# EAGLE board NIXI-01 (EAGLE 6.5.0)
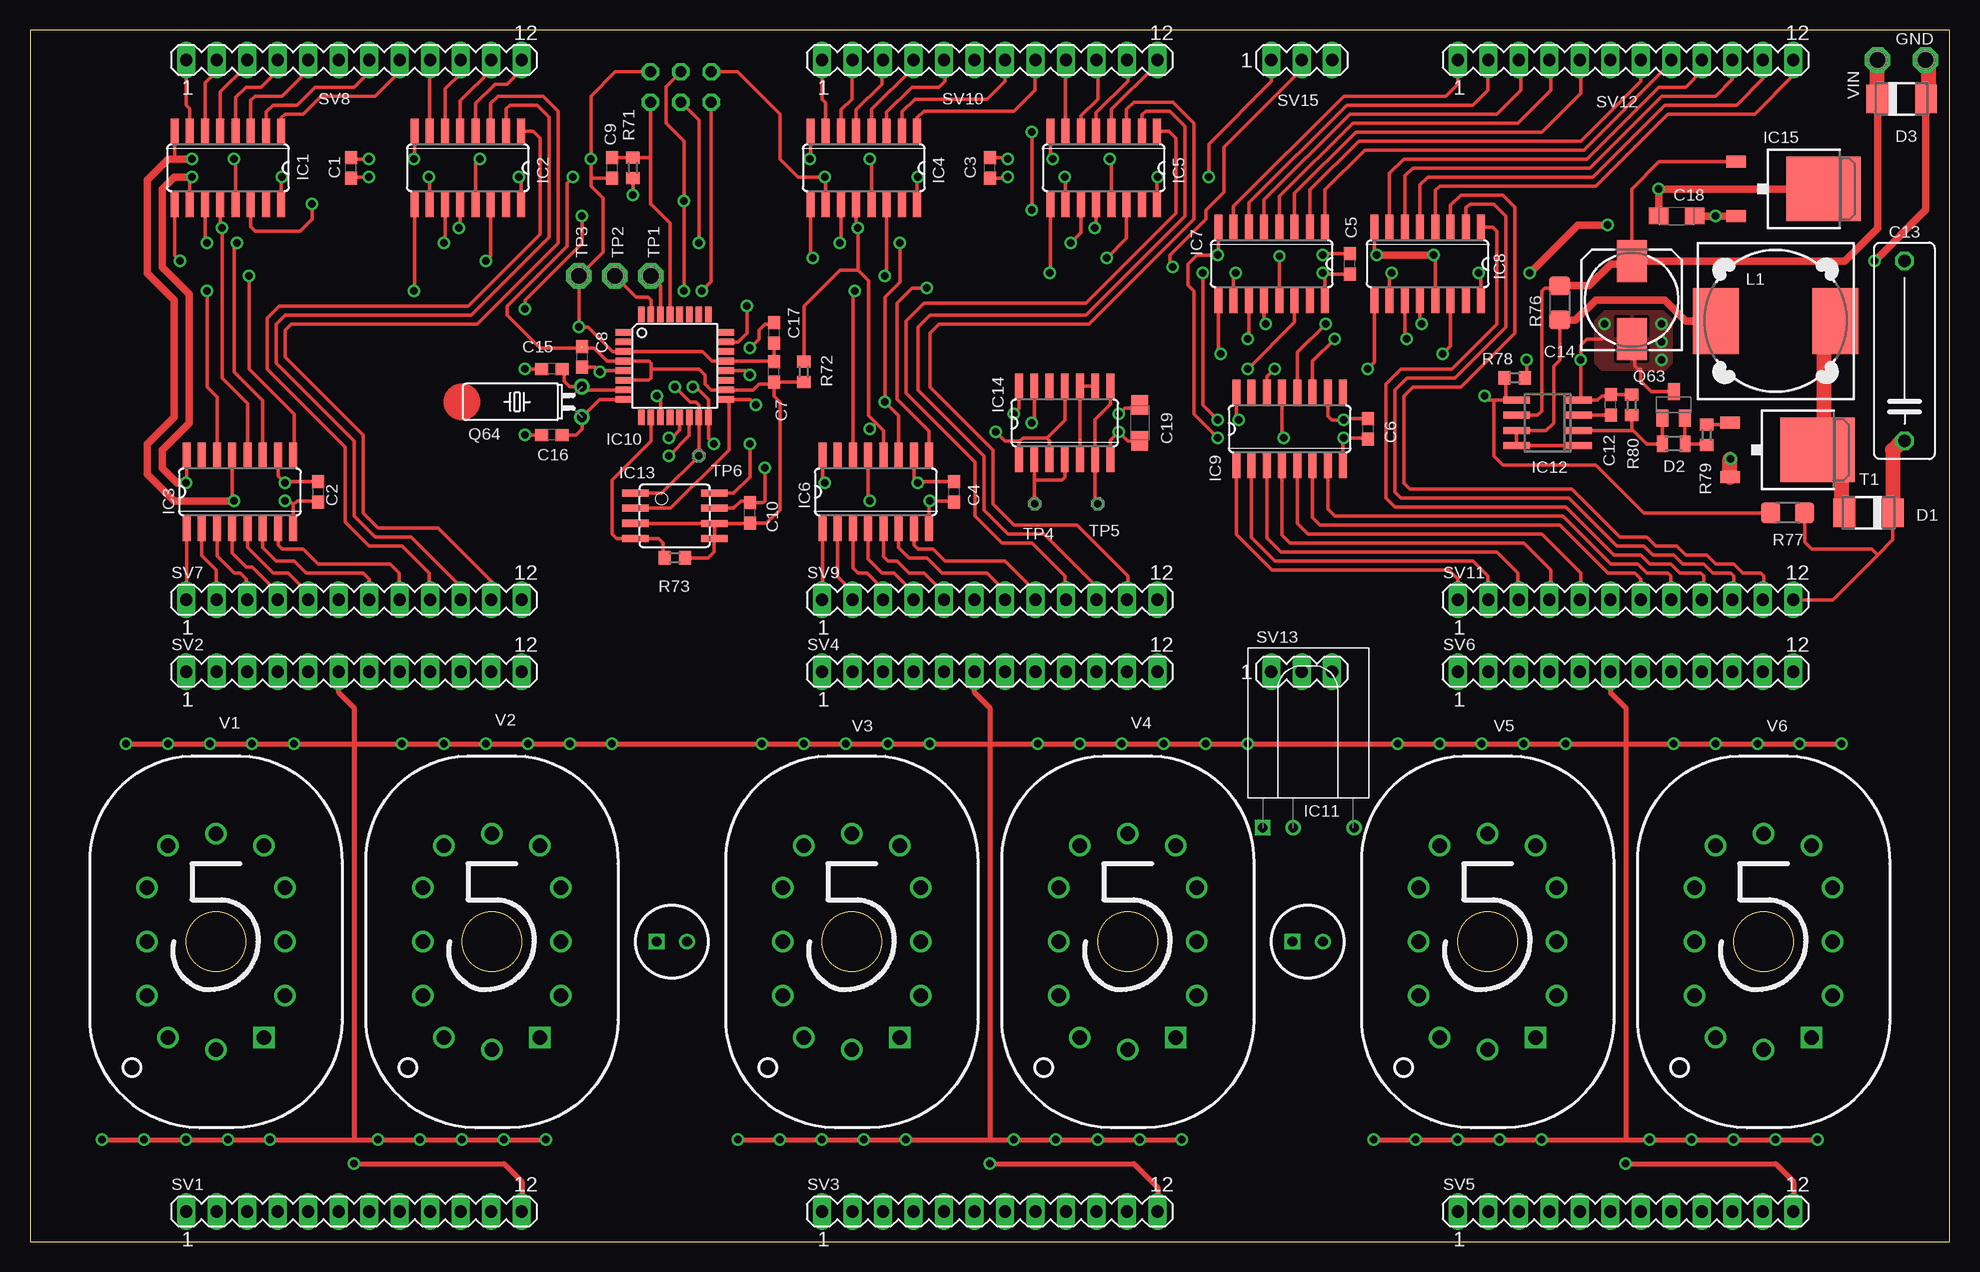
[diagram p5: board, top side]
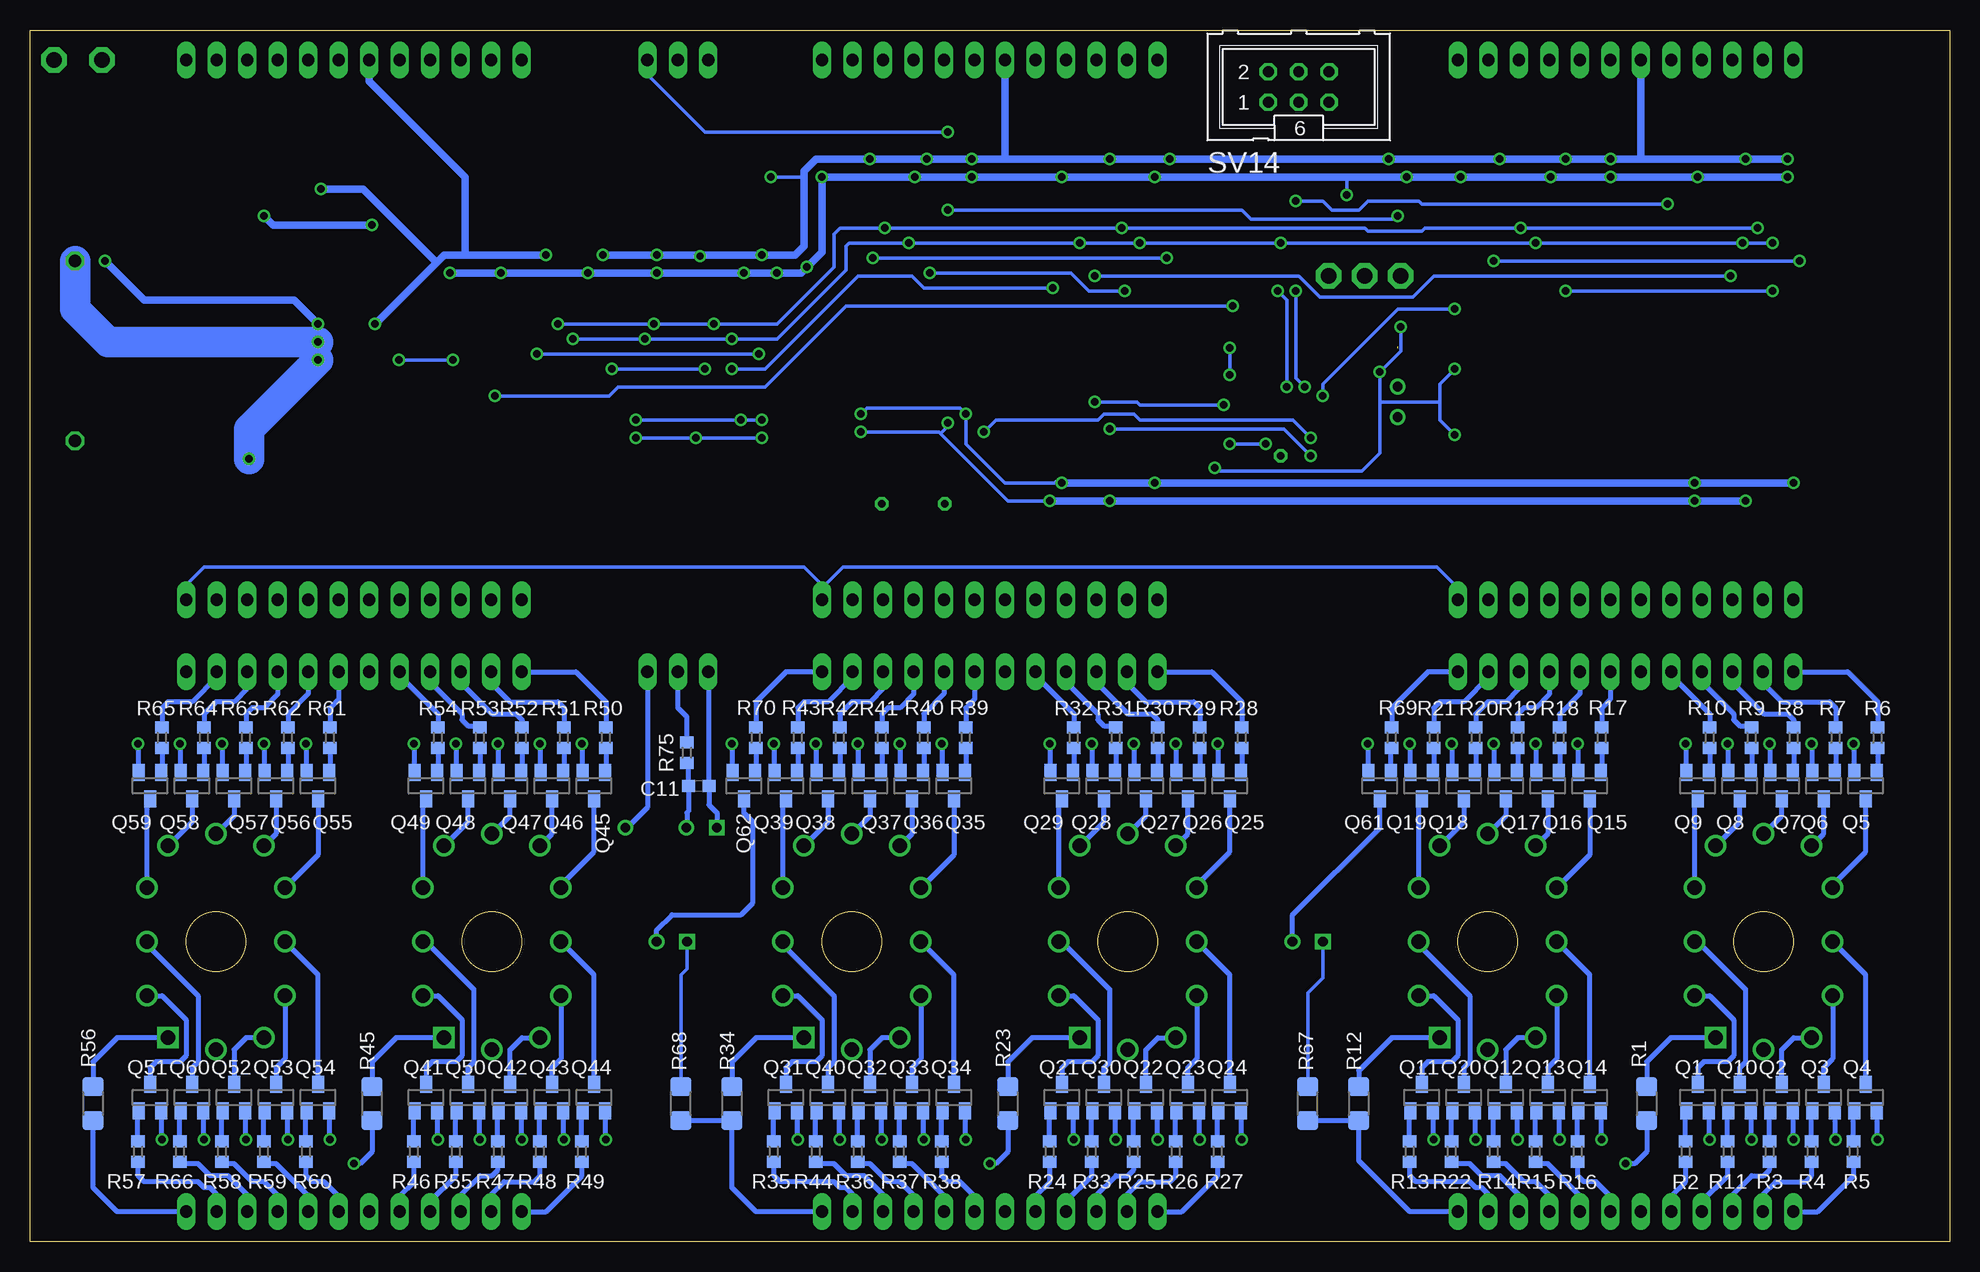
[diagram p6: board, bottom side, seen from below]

Size 160 x 101 mm. Coordinates in mm from the lower left corner, seen from the top.
Outline: 0,0 160,0 160,101 0,101 0,0
Copper layers (1*16): Top 0.035mm / dielectric 1.5mm / Bottom 0.035mm
Design rules "default *": minimum track width 0.3mm, minimum drill 0.6mm, track to track 0.35mm, track to pad 0.35mm, pad to pad 0.22mm, via to via 0.35mm, smd to smd 8mil, copper to edge 0.9mm, drill to drill 8mil, minimum pad ring 10mil, minimum via ring 8mil, stop-mask expansion 4mil, vias tented up to drill 0mil, thermal gap 10mil

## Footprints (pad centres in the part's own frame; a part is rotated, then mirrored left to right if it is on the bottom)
C0603 = smd 1.1 x 1: 1 -0.85,0; 2 0.85,0
C150-054X183 = drill 1.016 octagon: 1 -7.493,0; 2 7.493,0
153CLV-0810 = smd 3.5 x 2.5: + 3.25,0; - -3.25,0
SMC_A = smd 1.6 x 1.4: + -1.5,0; - 1.5,0
DO-214AC = smd 1.8 x 2.4: A 2.025,0; C -2.025,0
MICROMELF-W = smd 0.9 x 1.4: A 0.95,0; C -0.95,0
P1-13 = drill 1.321 pad 2.159 octagon: TP 0,0
SO16 = smd 0.66 x 2.032: 1 -4.445,-3.073; 2 -3.175,-3.073; 3 -1.905,-3.073; 4 -0.635,-3.073; 5 0.635,-3.073; 6 1.905,-3.073; 7 3.175,-3.073; 8 4.445,-3.073; 9 4.445,3.073; 10 3.175,3.073; 11 1.905,3.073; 12 0.635,3.073; 13 -0.635,3.073; 14 -1.905,3.073; 15 -3.175,3.073; 16 -4.445,3.073
TQFP32-08 = smd 1.27 x 0.559: 1 -4.293,2.8; 2 -4.293,2; 3 -4.293,1.2; 4 -4.293,0.4; 5 -4.293,-0.4; 6 -4.293,-1.2; 7 -4.293,-2; 8 -4.293,-2.8; 17 4.293,-2.8; 18 4.293,-2; 19 4.293,-1.2; 20 4.293,-0.4; 21 4.293,0.4; 22 4.293,1.2; 23 4.293,2; 24 4.293,2.8 | smd 0.559 x 1.27: 9 -2.8,-4.293; 10 -2,-4.293; 11 -1.2,-4.293; 12 -0.4,-4.293; 13 0.4,-4.293; 14 1.2,-4.293; 15 2,-4.293; 16 2.8,-4.293; 25 2.8,4.293; 26 2,4.293; 27 1.2,4.293; 28 0.4,4.293; 29 -0.4,4.293; 30 -1.2,4.293; 31 -2,4.293; 32 -2.8,4.293
TSOPXXXX_H = drill 0.8 square: 1 -3.74,0 | drill 0.8: 2 -1.2,0; 3 3.88,0
SO-08 = smd 0.6 x 2.2: 1 -1.905,-2.6; 2 -0.635,-2.6; 3 0.635,-2.6; 4 1.905,-2.6; 5 1.905,2.6; 6 0.635,2.6; 7 -0.635,2.6; 8 -1.905,2.6
8S2 = smd 0.6 x 2.2: 1 -1.905,-3.304; 2 -0.645,-3.304; 3 0.625,-3.304; 4 1.895,-3.304; 5 1.905,3.304; 6 0.635,3.304; 7 -0.635,3.304; 8 -1.905,3.304
SO14 = smd 0.66 x 2.032: 1 -3.81,-3.073; 2 -2.54,-3.073; 3 -1.27,-3.073; 4 0,-3.073; 5 1.27,-3.073; 6 2.54,-3.073; 7 3.81,-3.073; 8 3.81,3.073; 9 2.54,3.073; 10 1.27,3.073; 11 0,3.073; 12 -1.27,3.073; 13 -2.54,3.073; 14 -3.81,3.073
DPACK_1 = smd 1 x 1.6: 1 -2.28,-4.8; 2 2.28,-4.8 | smd 5.4 x 6.2: 3 0,2.5
DR125 = smd 3.85 x 5.5: 1 -4.975,0; 2 4.975,0
NEONLAMP_6X28 = drill 0.8 square: A -1.27,0 | drill 0.8: C 1.27,0
SOT23 = smd 1 x 1.4: 1 -0.95,-1.1; 2 0.95,-1.1; 3 0,1.1
SOT23-BEC = smd 1 x 1.4: B -0.95,-1.1; C 0,1.1; E 0.95,-1.1
TC38H = drill 0.813: 1 -1.27,0; 2 1.27,0
R1206 = smd 1.6 x 1.803: 1 -1.422,0; 2 1.422,0
R0603 = smd 1 x 1.1: 1 -0.85,0; 2 0.85,0
MA12-1 = drill 1.016 long: 1 -13.97,0; 2 -11.43,0; 3 -8.89,0; 4 -6.35,0; 5 -3.81,0; 6 -1.27,0; 7 1.27,0; 8 3.81,0; 9 6.35,0; 10 8.89,0; 11 11.43,0; 12 13.97,0
MA03-1 = drill 1.016 long: 1 -2.54,0; 2 0,0; 3 2.54,0
ML6 = drill 0.914 octagon: 1 -2.54,-1.27; 2 -2.54,1.27; 3 0,-1.27; 4 0,1.27; 5 2.54,-1.27; 6 2.54,1.27
P1-06 = drill 0.6 octagon: TP 0,0
NIXI_IN-12 = drill 1.2 square: 1 4,-8 | drill 1.2: 2 5.75,-4.5; 3 5.75,0; 4 5.75,4.5; 5 4,8; 6 0,9; 7 -4,8; 8 -5.75,4.5; 9 -5.75,0; 10 -5.75,-4.5; 11 -4,-8; 12 0,-9

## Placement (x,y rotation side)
C1  100n  [C0603]  26.75,89.5 90 top
C2  100n  [C0603]  24,62.5 270 top
C3  100n  [C0603]  80,89.5 90 top
C4  100n  [C0603]  77,62.5 270 top
C5  100n  [C0603]  110,81.5 90 top
C6  100n  [C0603]  111.5,67.75 270 top
C7  100n  [C0603]  62,72.5 90 top
C8  100n  [C0603]  46,73.75 270 top
C9  100n  [C0603]  48.5,89.5 270 top
C10  100n  [C0603]  60,60.75 90 top
C11  100n  [C0603]  104.25,38 0 bottom
C12  330p  [C0603]  131.75,69.75 90 top
C13  330n  [C150-054X183]  156.25,74.25 90 top
C14  100u  [153CLV-0810]  133.5,78.5 90 top
C15  22p  [C0603]  43.5,72.75 180 top
C16  22p  [C0603]  43.5,67.25 180 top
C17  100n  [C0603]  62,75.75 270 top
C18  2u2  [SMC_A]  137.25,85.5 180 top
C19  2u2  [SMC_A]  92.5,68.25 270 top
D1  BYG23M  [DO-214AC]  153.25,60.75 180 top
D2  LL4448  [MICROMELF-W]  137,66.5 180 top
D3  BYG23M  [DO-214AC]  156,95.25 0 top
GND  TPPAD1-13  [P1-13]  158,98.5 0 top
IC1  74HC595D  [SO16]  16.5,89.5 180 top
IC2  74HC595D  [SO16]  36.5,89.5 180 top
IC3  74HC595D  [SO16]  17.5,62.5 0 top
IC4  74HC595D  [SO16]  69.5,89.5 180 top
IC5  74HC595D  [SO16]  89.5,89.5 180 top
IC6  74HC595D  [SO16]  70.5,62.5 0 top
IC7  74HC595D  [SO16]  103.5,81.5 180 top
IC8  74HC595D  [SO16]  116.5,81.5 180 top
IC9  74HC595D  [SO16]  105,67.75 0 top
IC10  MEGA8-AI  [TQFP32-08]  53.75,73 0 top
IC11  TSOPXXXXH  [TSOPXXXX_H]  106.5,34.5 0 top
IC12  MC34063SO  [SO-08]  126.5,68.25 90 top
IC13  AT45DB321D-SU  [8S2]  53.75,60.5 270 top
IC14  74HC04D  [SO14]  86.25,68.25 0 top
IC15  LF33  [DPACK_1]  147,87.75 270 top
L1  68u  [DR125]  145.5,76.75 0 top
LMP1  [NEONLAMP_6X28]  53.5,25 0 top
LMP2  [NEONLAMP_6X28]  106.5,25 0 top
Q1  [SOT23]  21,12 0 bottom
Q2  [SOT23]  14,12 0 bottom
Q3  [SOT23]  10.5,12 0 bottom
Q4  [SOT23]  7,12 0 bottom
Q5  [SOT23]  7,38 180 bottom
Q6  [SOT23]  10.5,38 180 bottom
Q7  [SOT23]  14,38 180 bottom
Q8  [SOT23]  17.5,38 180 bottom
Q9  [SOT23]  21,38 180 bottom
Q10  [SOT23]  17.5,12 0 bottom
Q11  [SOT23]  44,12 0 bottom
Q12  [SOT23]  37,12 0 bottom
Q13  [SOT23]  33.5,12 0 bottom
Q14  [SOT23]  30,12 0 bottom
Q15  [SOT23]  30,38 180 bottom
Q16  [SOT23]  33.5,38 180 bottom
Q17  [SOT23]  37,38 180 bottom
Q18  [SOT23]  40.5,38 180 bottom
Q19  [SOT23]  44,38 180 bottom
Q20  [SOT23]  40.5,12 0 bottom
Q21  [SOT23]  74,12 0 bottom
Q22  [SOT23]  67,12 0 bottom
Q23  [SOT23]  63.5,12 0 bottom
Q24  [SOT23]  60,12 0 bottom
Q25  [SOT23]  60,38 180 bottom
Q26  [SOT23]  63.5,38 180 bottom
Q27  [SOT23]  67,38 180 bottom
Q28  [SOT23]  70.5,38 180 bottom
Q29  [SOT23]  74,38 180 bottom
Q30  [SOT23]  70.5,12 0 bottom
Q31  [SOT23]  97,12 0 bottom
Q32  [SOT23]  90,12 0 bottom
Q33  [SOT23]  86.5,12 0 bottom
Q34  [SOT23]  83,12 0 bottom
Q35  [SOT23]  83,38 180 bottom
Q36  [SOT23]  86.5,38 180 bottom
Q37  [SOT23]  90,38 180 bottom
Q38  [SOT23]  93.5,38 180 bottom
Q39  [SOT23]  97,38 180 bottom
Q40  [SOT23]  93.5,12 0 bottom
Q41  [SOT23]  127,12 0 bottom
Q42  [SOT23]  120,12 0 bottom
Q43  [SOT23]  116.5,12 0 bottom
Q44  [SOT23]  113,12 0 bottom
Q45  [SOT23]  113,38 180 bottom
Q46  [SOT23]  116.5,38 180 bottom
Q47  [SOT23]  120,38 180 bottom
Q48  [SOT23]  123.5,38 180 bottom
Q49  [SOT23]  127,38 180 bottom
Q50  [SOT23]  123.5,12 0 bottom
Q51  [SOT23]  150,12 0 bottom
Q52  [SOT23]  143,12 0 bottom
Q53  [SOT23]  139.5,12 0 bottom
Q54  [SOT23]  136,12 0 bottom
Q55  [SOT23]  136,38 180 bottom
Q56  [SOT23]  139.5,38 180 bottom
Q57  [SOT23]  143,38 180 bottom
Q58  [SOT23]  146.5,38 180 bottom
Q59  [SOT23]  150,38 180 bottom
Q60  [SOT23]  146.5,12 0 bottom
Q61  [SOT23]  47.5,38 180 bottom
Q62  [SOT23]  100.5,38 180 bottom
Q63  BC856A  [SOT23-BEC]  137,69.75 0 top
Q64  32.768kHz  [TC38H]  46,70 90 top
R1  15k  [R1206]  25.25,11.5 90 bottom
R2  10k  [R0603]  22,7.5 90 bottom
R3  10k  [R0603]  15,7.5 90 bottom
R4  10k  [R0603]  11.5,7.5 90 bottom
R5  10k  [R0603]  8,7.5 90 bottom
R6  10k  [R0603]  6,42 270 bottom
R7  10k  [R0603]  9.5,42 270 bottom
R8  10k  [R0603]  13,42 270 bottom
R9  10k  [R0603]  16.5,42 270 bottom
R10  10k  [R0603]  20,42 270 bottom
R11  10k  [R0603]  18.5,7.5 90 bottom
R12  15k  [R1206]  49.25,11.5 90 bottom
R13  10k  [R0603]  45,7.5 90 bottom
R14  10k  [R0603]  38,7.5 90 bottom
R15  10k  [R0603]  34.5,7.5 90 bottom
R16  10k  [R0603]  31,7.5 90 bottom
R17  10k  [R0603]  29,42 270 bottom
R18  10k  [R0603]  32.5,42 270 bottom
R19  10k  [R0603]  36,42 270 bottom
R20  10k  [R0603]  39.5,42 270 bottom
R21  10k  [R0603]  43,42 270 bottom
R22  10k  [R0603]  41.5,7.5 90 bottom
R23  15k  [R1206]  78.5,11.5 90 bottom
R24  10k  [R0603]  75,7.5 90 bottom
R25  10k  [R0603]  68,7.5 90 bottom
R26  10k  [R0603]  64.5,7.5 90 bottom
R27  10k  [R0603]  61,7.5 90 bottom
R28  10k  [R0603]  59,42 270 bottom
R29  10k  [R0603]  62.5,42 270 bottom
R30  10k  [R0603]  66,42 270 bottom
R31  10k  [R0603]  69.5,42 270 bottom
R32  10k  [R0603]  73,42 270 bottom
R33  10k  [R0603]  71.5,7.5 90 bottom
R34  15k  [R1206]  101.5,11.5 90 bottom
R35  10k  [R0603]  98,7.5 90 bottom
R36  10k  [R0603]  91,7.5 90 bottom
R37  10k  [R0603]  87.5,7.5 90 bottom
R38  10k  [R0603]  84,7.5 90 bottom
R39  10k  [R0603]  82,42 270 bottom
R40  10k  [R0603]  85.5,42 270 bottom
R41  10k  [R0603]  89,42 270 bottom
R42  10k  [R0603]  92.5,42 270 bottom
R43  10k  [R0603]  96,42 270 bottom
R44  10k  [R0603]  94.5,7.5 90 bottom
R45  15k  [R1206]  131.5,11.5 90 bottom
R46  10k  [R0603]  128,7.5 90 bottom
R47  10k  [R0603]  121,7.5 90 bottom
R48  10k  [R0603]  117.5,7.5 90 bottom
R49  10k  [R0603]  114,7.5 90 bottom
R50  10k  [R0603]  112,42 270 bottom
R51  10k  [R0603]  115.5,42 270 bottom
R52  10k  [R0603]  119,42 270 bottom
R53  10k  [R0603]  122.5,42 270 bottom
R54  10k  [R0603]  126,42 270 bottom
R55  10k  [R0603]  124.5,7.5 90 bottom
R56  15k  [R1206]  154.75,11.5 90 bottom
R57  10k  [R0603]  151,7.5 90 bottom
R58  10k  [R0603]  144,7.5 90 bottom
R59  10k  [R0603]  140.5,7.5 90 bottom
R60  10k  [R0603]  137,7.5 90 bottom
R61  10k  [R0603]  135,42 270 bottom
R62  10k  [R0603]  138.5,42 270 bottom
R63  10k  [R0603]  142,42 270 bottom
R64  10k  [R0603]  145.5,42 270 bottom
R65  10k  [R0603]  149,42 270 bottom
R66  10k  [R0603]  147.5,7.5 90 bottom
R67  220k  [R1206]  53.5,11.5 270 bottom
R68  220k  [R1206]  105.75,11.5 270 bottom
R69  10k  [R0603]  46.5,42 90 bottom
R70  10k  [R0603]  99.5,42 90 bottom
R71  10k  [R0603]  50.25,89.5 270 top
R72  10k  [R0603]  64.5,72.5 270 top
R73  10k  [R0603]  53.75,57 0 top
R75  100  [R0603]  105.25,40.75 270 bottom
R76  0R22  [R1206]  127.5,78.25 90 top
R77  1M  [R1206]  146.5,60.75 0 top
R78  6k8  [R0603]  123.75,72 180 top
R79  33R  [R0603]  139.75,67.25 270 top
R80  1k  [R0603]  133.5,69.75 90 top
SV1  [MA12-1]  27,2.5 0 top
SV2  [MA12-1]  27,47.5 0 top
SV3  [MA12-1]  80,2.5 0 top
SV4  [MA12-1]  80,47.5 0 top
SV5  [MA12-1]  133,2.5 0 top
SV6  [MA12-1]  133,47.5 0 top
SV7  [MA12-1]  27,53.5 0 top
SV8  [MA12-1]  27,98.5 0 top
SV9  [MA12-1]  80,53.5 0 top
SV10  [MA12-1]  80,98.5 0 top
SV11  [MA12-1]  133,53.5 0 top
SV12  [MA12-1]  133,98.5 0 top
SV13  [MA03-1]  106,47.5 0 top
SV14  [ML6]  54.25,96.25 0 bottom
SV15  [MA03-1]  106,98.5 0 top
T1  IRFR 13N20D  [DPACK_1]  146.5,66 270 top
TP1  TPPAD1-13  [P1-13]  51.75,80.5 0 top
TP2  TPPAD1-13  [P1-13]  48.75,80.5 0 top
TP3  TPPAD1-13  [P1-13]  45.75,80.5 0 top
TP4  [P1-06]  83.75,61.5 0 top
TP5  [P1-06]  89,61.5 0 top
TP6  [P1-06]  55.75,65.5 0 top
U$1  [A4L-LOC]  not placed on the board
V1  NIXI-IN-12  [NIXI_IN-12]  15.5,25 0 top
V2  NIXI-IN-12  [NIXI_IN-12]  38.5,25 0 top
V3  NIXI-IN-12  [NIXI_IN-12]  68.5,25 0 top
V4  NIXI-IN-12  [NIXI_IN-12]  91.5,25 0 top
V5  NIXI-IN-12  [NIXI_IN-12]  121.5,25 0 top
V6  NIXI-IN-12  [NIXI_IN-12]  144.5,25 0 top
VIN  TPPAD1-13  [P1-13]  154,98.5 0 top

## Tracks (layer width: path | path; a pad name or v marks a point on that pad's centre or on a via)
+3V3  (via drill 0.6)  (1 unrouted)
  Top 0.305: 41,86.48 IC2.16 40.95,88.56 v40.75,88.75 | C1.1 26.6,88.65 26.5,88.75 | IC1.16 20.95,88.69 v21,88.75 | 26.65,88.75 C1.1 | v28.25,88.75 26.85,88.75 C1.1 | IC2.10 33.33,88.67 v33.25,88.75 | IC8.16 120.94,80.56 v120.75,80.75 | IC8.10 113.33,80.58 v113.5,80.75 | IC5.10 86.33,88.67 v86.25,88.75 | IC5.16 93.94,88.69 v94,88.75 | IC4.16 73.94,88.69 v74,88.75 | C3.1 81.4,88.65 v81.5,88.75 | IC1.10 13.32,88.58 v13.5,88.75 | C2.1 21.35,63.35 v21.25,63.25 20.68,63.83 IC3.10 | C6.1 109.6,68.6 v109.5,68.5 108.5,68.5 108.17,68.83 IC9.10 | IC9.16 100.56,68.69 v100.75,68.5 | IC6.16 66.06,63.45 v66.25,63.25 | IC6.10 73.67,63.58 v74,63.25 74.1,63.35 C4.1 | IC4.10 66.33,88.67 v66.25,88.75 64,88.75 62.5,90.25 62.5,94 58.98,97.52 SV14.2 | IC3.16 13.05,63.3 v13,63.25 | v99,68.5 97.75,69.75 v97.75,80.75 | IC7.10 100.33,80.58 v100.5,80.75 | IC7.16 107.94,80.56 v107.75,80.75 107.85,80.65 C5.1 | SV15.2 106,97.75 99.5,91.25 99.5,87.5 98,86 98,85.25 95,82.25 95,81.5 v95.25,81.25 | C7.1 61.85,71.5 60.75,71.5 60.25,71 IC10.18 56.75,71 56.25,71.5 56.25,72.25 55.75,72.75 51.75,72.75 | C7.1 R72.2 | IC10.6 51.55,71.8 51.75,72 51.75,72.75 | 51.75,72.75 51.75,73.25 51.6,73.4 IC10.4 48.1,73.4 47,74.5 46.1,74.5 C8.1 | v45.25,88.75 44.75,88.25 44.75,83 39.75,78 39.75,77.25 42.5,74.5 46,74.5 | R71.2 v50.25,87.25 | IC13.3 57.03,59.88 arc-45 IC13.6 | IC13.6 IC13.5 57,58.54 57,57.5 56.5,57 R73.2 | IC13.6 59.92,59.87 arc45 C10.1 61.4,59.9 62.5,61 62.5,70 62,70.5 C7.1 | v90.75,69 91.25,69.5 92.25,69.5 C19.+ | IC14.14 82.44,69.44 v82,69 | 142.17,85.5 IC15.2
  Top 0.61: v13,63.25 12.25,63.25 11,64.5 11,66 13.25,68.25 13.25,79 11,81.25 11,87.75 12,88.75 v13.5,88.75 | v125,80.75 129,84.75 v131.5,84.75 | 142.17,85.5 v140.5,85.5 C18.+
  Bottom 0.305: v109.5,68.5 v100.75,68.5 v99,68.5 | v50.25,87.25 50.25,88.75 | v74,63.25 74.1,63.35 74.5,63.35 74.6,63.25 78.75,63.25 82,66.5 v82,69 82.5,69.5 90.25,69.5 v90.75,69
  Bottom 0.61: v13.5,88.75 v21,88.75 v28.25,88.75 v33.25,88.75 v40.75,88.75 v45.25,88.75 50.25,88.75 v66.25,88.75 v74,88.75 v81.5,88.75 v86.25,88.75 v94,88.75 94,82.5 v95.25,81.25 95.75,80.75 v97.75,80.75 v100.5,80.75 v107.75,80.75 v113.5,80.75 v120.75,80.75 v125,80.75 | v13,63.25 v21.25,63.25 v66.25,63.25 v74,63.25 | v131.5,84.75 139.75,84.75 v140.5,85.5
+12V
  Top 0.305: IC12.6 125.64,68.89 126,69.25 126,79.25 126.25,79.5 127.33,79.5 R76.2 | 133.25,81.5 C14.+ 133.5,87.75 135.78,90.03 IC15.1 | 154,95.22 D3.C
  Top 0.61: R76.2 129.92,79.67 131.75,81.5 133.25,81.5 | C14.+ 151.25,81.75 154,84.5 154,95.22
  Top 1.27: D3.C 153.97,98.47 VIN.TP
CS_SH  (via drill 0.6)
  Top 0.305: IC1.12 15.87,84.64 v16,84.5 16,72 18.14,69.86 IC3.12 | IC5.12 88.86,84.61 v88.75,84.5 | IC4.12 68.86,84.64 v69,84.5 69,81 | IC2.12 35.87,84.61 v35.75,84.5 | IC8.12 115.86,76.64 v116,76.5 | IC7.12 102.86,76.64 v103,76.5 | 70.5,68.25 71.14,67.61 IC6.12 | 70.5,68.25 69.89,68.86 69.89,80.11 69,81 | IC9.12 105.64,74.14 v108,76.5 | R72.1 64.5,78 67.5,81 69,81 | v70,67.75 70.5,68.25 | IC10.14 54.95,67.2 v53.25,65.5
  Bottom 0.305: v16,84.5 v35.75,84.5 43.75,84.5 44,84.25 48.5,84.25 48.75,84.5 v69,84.5 v88.75,84.5 92.5,84.5 93,84 93,81.25 97.75,76.5 v103,76.5 v108,76.5 v116,76.5 | v53.25,65.5 55.5,67.75 v70,67.75
GND  (via drill 0.6)
  Top 0.305: IC3.8 21.95,61.45 | 21.95,61.45 22.25,61.75 23.9,61.75 C2.2 | IC1.13 17.14,90.11 v17,90.25 | IC8.8 112.06,82.44 v112.25,82.25 | IC8.13 117.14,82.11 v117,82.25 | IC7.8 99.06,82.31 v99,82.25 97.25,82.25 96.5,81.5 96.5,79.75 97,79.25 97,69 v99,67 | IC7.13 v104.14,82.14 | IC5.13 90.14,90.11 v90,90.25 | IC5.8 85.06,90.44 v85.25,90.25 | IC4.13 70.14,90.11 v70,90.25 | IC4.8 65.06,90.31 v65,90.25 | IC2.13 37.13,89.89 v37.5,90.25 | IC2.8 32.05,90.31 v32,90.25 | C1.2 26.75,90.25 v28.25,90.25 | C5.2 107.85,82.35 v107.75,82.25 | C3.2 81.4,90.35 v81.5,90.25 | IC3.13 16.86,61.88 v17,61.75 | v21.25,61.75 21.64,61.75 21.95,61.45 | IC9.13 104.36,67.14 v104.5,67 | IC6.13 69.86,61.88 v70,61.75 | IC6.8 74.94,61.7 v75,61.75 76.9,61.75 C4.2 | 131.71,70.31 C12.2 | Q63.C 135.15,70.85 134.25,71.75 134.25,72.75 134,72.75 133.75,73 133.75,75 C14.- 133.75,75.5 | 141.7,65.2 v141.75,65.25 | 133.5,76.5 133.5,76 | IC1.8 12.05,90.31 12,90.25 | 131,75.25 129.75,75.25 129.25,74.75 v129.25,73.5 129.25,70.25 129.19,70.25 IC12.4 130.66,70.16 131,70.5 131.65,70.5 C12.2 | R80.2 C12.2 | SV15.1 103.46,96.71 98.25,91.5 v98.25,88.75 | C17.2 C7.2 61.95,73.4 IC10.21 56.85,73.4 56.05,74.2 IC10.3 48.55,74.2 46.5,76.25 v45.75,76.25 TP3.TP 47.75,82.5 47.75,87 46.75,88 46.75,88.75 | 46.3,72.6 C8.2 47.1,72.9 v47.5,72.5 47.6,72.6 IC10.5 | 46.75,88.75 v46.75,90.25 46.75,95.5 48.77,97.52 SV14.6 | v41.25,67.25 C16.2 | C15.2 v41.25,72.75 | C9.2 46.98,88.65 arc-45 46.76,88.74 46.75,88.75 | IC13.7 58.5,61.13 arc45 58.73,61.23 59.25,61.75 59.72,61.75 arc-45 59.94,61.66 C10.2 61.1,61.6 61.25,61.75 v61.25,64.5 | IC14.7 90.06,66.81 v90.75,67.5 91.5,66.75 C19.-
  Top 0.305: IC14.13 83.71,68.46 v83.5,68.25 | IC9.8 109.44,66.94 v109.5,67 111.25,67 111.35,66.9 C6.2 | v124.75,73.5 124.75,72.15 R78.1
  Top 0.61: v13.5,90.25 12,90.25 11.5,90.25 9.75,88.5 9.75,80.75 12,78.5 12,68.75 9.75,66.5 9.75,64 12,61.75 v17,61.75 | 134.25,75 133.75,75.5 | 158.25,95.47 D3.A 158.03,86.03 v153.75,81.75 | 134,76.5 133.5,76 C14.- | v112.25,82.25 v117,82.25 | IC15.3 v135.75,87.75 C18.-
  Top 1.27: T1.2 141.7,65.2 | 158.25,95.47 158.25,98.25 GND.TP
  Bottom 0.305: 25.73,90.27 25.75,90.25 | v104.14,82.14 104.25,82.25 | 78.73,90.27 78.75,90.25 | 105.73,82.27 105.75,82.25 | v109.5,67 v104.5,67 v99,67 | v98.25,88.75 95.5,88.75 | 47.5,70 42.5,70 | 42.5,70 42.5,71.5 v41.25,72.75 | 42.5,70 42.5,68.5 v41.25,67.25 | 47.5,70 47.5,65.75 49,64.25 61,64.25 v61.25,64.5 | 47.5,70 v47.5,72.5 45.75,74.25 v45.75,76.25 | v90.75,67.5 84.25,67.5 84.12,67.38 | 84.12,67.38 78.5,61.75 v75,61.75 | v83.5,68.25 83.5,68 84.12,67.38 | v124.75,73.5 v129.25,73.5
  Bottom 0.61: v13.5,90.25 v17,90.25 25.75,90.25 v28.25,90.25 v32,90.25 v37.5,90.25 v46.75,90.25 v65,90.25 v70,90.25 78.75,90.25 v81.5,90.25 v85.25,90.25 v90,90.25 94.5,90.25 95.5,89.25 95.5,88.75 95.5,83 96.25,82.25 v99,82.25 104.25,82.25 105.75,82.25 v107.75,82.25 v112.25,82.25 | SV8.6 25.73,90.27 | SV10.6 78.73,90.27 | v17,61.75 v21.25,61.75 v70,61.75 v75,61.75 | SV12.6 131.73,96.73 123.75,88.75 123.75,82.25 | v153.75,81.75 150.5,78.5 138,78.5 v136,76.5 | 123.75,82.25 125.5,82.25 126.12,81.62 | 126.12,81.62 v131.25,76.5 | 123.75,82.25 v117,82.25 | v135.75,87.75 132.25,87.75 126.12,81.62
  Bottom 2.54: v141.75,65.25 141.75,67.75 v136,73.5 | v136,75 153.5,75 156.25,77.75 C13.2
  pour Top: 131.25,77.5 136.25,77.5 136.75,77 136.75,73.25 136.25,72.75 131,72.75 130.5,73.25 130.5,76.75
GNDA  (via drill 0.6)
  Top 0.406: 27,41.5 27,44.5 25.73,45.77 SV2.6 | 27,41.5 27,8.5 | v6,8.5 v9.5,8.5 v13,8.5 v16.5,8.5 v20,8.5 27,8.5 | 27,8.5 v29,8.5 v32.5,8.5 v36,8.5 v39.5,8.5 v43,8.5 | v8,41.5 v11.5,41.5 v15,41.5 v18.5,41.5 v22,41.5 27,41.5 | 27,41.5 v31,41.5 v34.5,41.5 v38,41.5 v41.5,41.5 v45,41.5 v48.5,41.5 v61,41.5 v64.5,41.5 v68,41.5 v71.5,41.5 v75,41.5 80,41.5 | 80,41.5 80,44.5 78.73,45.77 SV4.6 | 80,41.5 80,8.5 | v59,8.5 v62.5,8.5 v66,8.5 v69.5,8.5 v73,8.5 80,8.5 | 80,8.5 v82,8.5 v85.5,8.5 v89,8.5 v92.5,8.5 v96,8.5 | 80,41.5 v84,41.5 v87.5,41.5 v91,41.5 v94.5,41.5 v98,41.5 v101.5,41.5 v114,41.5 v117.5,41.5 v121,41.5 v124.5,41.5 v128,41.5 133,41.5 | SV6.6 131.73,45.77 133,44.5 133,41.5 | 133,41.5 133,8.5 | v112,8.5 v115.5,8.5 v119,8.5 v122.5,8.5 v126,8.5 133,8.5 | 133,8.5 v135,8.5 v138.5,8.5 v142,8.5 v145.5,8.5 v149,8.5 | 133,41.5 v137,41.5 v140.5,41.5 v144,41.5 v147.5,41.5 v151,41.5
  Bottom 0.406: Q5.2 7.95,41.45 v8,41.5 | Q6.2 11.45,41.45 v11.5,41.5 | Q7.2 14.95,41.45 v15,41.5 | Q8.2 18.45,41.45 v18.5,41.5 | Q9.2 21.95,41.45 v22,41.5 | Q15.2 30.95,41.45 v31,41.5 | Q16.2 34.45,41.45 v34.5,41.5 | Q17.2 37.95,41.45 v38,41.5 | Q18.2 41.45,41.45 v41.5,41.5 | Q19.2 44.95,41.45 v45,41.5 | Q61.2 48.45,41.45 v48.5,41.5 | Q25.2 60.95,41.45 v61,41.5 | Q26.2 64.45,41.45 v64.5,41.5 | Q27.2 67.95,41.45 v68,41.5 | Q28.2 71.45,41.45 v71.5,41.5 | Q29.2 74.95,41.45 v75,41.5 | Q35.2 83.95,41.45 v84,41.5 | Q36.2 87.45,41.45 v87.5,41.5 | Q37.2 90.95,41.45 v91,41.5 | Q38.2 94.45,41.45 v94.5,41.5 | Q39.2 97.95,41.45 v98,41.5 | Q62.2 101.45,41.45 v101.5,41.5 | Q45.2 113.95,41.45 v114,41.5 | Q46.2 117.45,41.45 v117.5,41.5 | Q47.2 120.95,41.45 v121,41.5 | Q48.2 124.45,41.45 v124.5,41.5 | Q49.2 127.95,41.45 v128,41.5 | Q55.2 136.95,41.45 v137,41.5 | Q56.2 140.45,41.45 v140.5,41.5 | Q57.2 143.95,41.45 v144,41.5 | Q58.2 147.45,41.45 v147.5,41.5 | Q59.2 150.95,41.45 v151,41.5 | Q51.2 149.05,8.55 v149,8.5 | Q60.2 145.55,8.55 v145.5,8.5 | Q52.2 142.05,8.55 v142,8.5 | Q53.2 138.55,8.55 v138.5,8.5 | Q54.2 135.05,8.55 v135,8.5 | Q41.2 126.05,8.55 v126,8.5 | Q50.2 122.55,8.55 v122.5,8.5 | Q42.2 119.05,8.55 v119,8.5 | Q43.2 115.55,8.55 v115.5,8.5 | Q44.2 112.05,8.55 v112,8.5 | Q31.2 96.05,8.55 v96,8.5 | Q40.2 92.55,8.55 v92.5,8.5 | Q32.2 89.05,8.55 v89,8.5 | Q33.2 85.55,8.55 v85.5,8.5 | Q34.2 82.05,8.55 v82,8.5 | Q21.2 73.05,8.55 v73,8.5 | Q30.2 69.55,8.55 v69.5,8.5 | Q22.2 66.05,8.55 v66,8.5 | Q23.2 62.55,8.55 v62.5,8.5 | Q24.2 59.05,8.55 v59,8.5 | Q11.2 43.05,8.55 v43,8.5 | Q20.2 39.55,8.55 v39.5,8.5 | Q12.2 36.05,8.55 v36,8.5 | Q13.2 32.55,8.55 v32.5,8.5 | Q14.2 29.05,8.55 v29,8.5
  Bottom 0.406: Q1.2 20.05,8.55 v20,8.5 | Q10.2 16.55,8.55 v16.5,8.5 | Q2.2 13.05,8.55 v13,8.5 | Q3.2 9.55,8.55 v9.5,8.5 | Q4.2 6.05,8.55 v6,8.5
MISO  (via drill 0.6)
  Top 0.305: SV14.1 56.79,80.04 v56,79.25 | v55.25,71.25 55.5,71.25 56.55,70.2 IC10.16 56.55,66.95 v57,66.5 | v60,66.5 60,63.75 58.66,62.41 IC13.8
  Bottom 0.305: v56,79.25 55.25,78.5 v55.25,71.25 | v57,66.5 v60,66.5
MOSI  (via drill 0.6)
  Top 0.305: IC1.14 18.41,84.59 18.75,84.25 22.5,84.25 23.5,85.25 v23.5,86.5 | SV14.4 53,96.27 53,93.25 54.5,91.75 v54.5,86.75 v54.5,79.25 | IC13.1 52.66,62.41 TP6.TP IC10.15 55.75,69.75 55.5,70 55,70 v53.75,71.25
  Bottom 0.305: v23.5,86.5 44,86.5 44.25,86.75 48.5,86.75 49.25,86 51.5,86 52.25,86.75 v54.5,86.75 | v54.5,79.25 54.5,72 v53.75,71.25
N$1
  Bottom 0.406: V1.1 23.25,17 25.25,15 R1.2
N$2
  Bottom 0.406: V1.2 20,20.5 18,18.5 18,15.5 18.5,15 20.5,15 21,14.5 Q1.3
N$3
  Bottom 0.406: Q2.3 14,16 13,17 V1.11
N$4
  Bottom 0.406: Q3.3 10.5,14.5 9.75,15.25 V1.10
N$5
  Bottom 0.406: Q4.3 7,22.25 V1.9
N$6
  Bottom 0.406: V1.8 9.75,29.75 7,32.5 Q5.3
N$7
  Bottom 0.406: V1.7 10.5,34 Q6.3
N$8
  Bottom 0.406: V1.6 14,35.5 Q7.3
N$9
  Bottom 0.406: V1.5 17.5,35 Q8.3
N$10
  Bottom 0.406: V1.4 21.25,36.65 Q9.3
N$11
  Bottom 0.406: V1.3 21,25 17,21 17,15 17.5,14.5 Q10.3
N$12
  Bottom 0.406: R3.2 15.05,8.4 15.05,10.8 Q2.1
N$13
  Bottom 0.406: R4.2 11.55,8.4 11.55,10.8 Q3.1
N$14
  Bottom 0.406: R5.2 8.05,8.4 8.05,10.8 Q4.1
N$15
  Bottom 0.406: R6.2 5.95,41.1 5.95,39.1 Q5.1
N$16
  Bottom 0.406: R7.2 9.45,41.1 9.45,39.1 Q6.1
N$17
  Bottom 0.406: R8.2 12.95,41.1 12.95,39.1 Q7.1
N$18
  Bottom 0.406: R9.2 16.45,41.1 16.45,39.1 Q8.1
N$19
  Bottom 0.406: R10.2 19.95,41.1 19.95,39.1 Q9.1
N$20
  Bottom 0.406: R11.2 18.55,8.4 18.55,10.8 Q10.1
N$21
  Bottom 0.406: R2.2 22.05,8.4 22.05,10.8 Q1.1
N$22
  Bottom 0.406: SV1.1 11,2.5 8,5.5 R5.1
N$23
  Bottom 0.406: SV1.2 15.57,3.93 14.5,5 12,5 11.5,5.5 R4.1
N$24
  Bottom 0.406: SV1.3 18.11,3.89 16.5,5.5 15.5,5.5 15,6 R3.1
N$25
  Bottom 0.406: SV1.4 20.65,3.35 18.5,5.5 R11.1
N$26
  Bottom 0.406: SV1.5 23.19,3.81 22,5 R2.1
N$27  (via drill 0.6)
  Top 0.305: IC2.14 38.41,82.16 v38,81.75 | IC1.9 12.05,82.19 v12.5,81.75
  Bottom 0.305: v38,81.75 v12.5,81.75
N$28
  Bottom 0.406: SV2.1 8.5,47.5 6,45 R6.1
N$29
  Bottom 0.406: SV2.2 15.57,46.57 14,45 10,45 9.5,44.5 R7.1
N$30
  Bottom 0.406: SV2.3 18.11,46.61 15.5,44 13.5,44 13,43.5 R8.1
N$31
  Bottom 0.406: SV2.4 20.65,46.65 18,44 18,43.5 17.5,43 16.65,43 R9.1
N$32
  Bottom 0.406: SV2.5 23.19,47.19 20,44 R10.1
N$33
  Bottom 0.406: V2.1 46.5,17 49.25,14.25 R12.2
N$34
  Bottom 0.406: V2.2 43,20.5 41,18.5 41,15.5 41.5,15 43.5,15 44,14.5 Q11.3
N$35
  Bottom 0.406: V2.11 36,17 37,16 Q12.3
N$36
  Bottom 0.406: V2.10 32.75,15.25 33.5,14.5 Q13.3
N$37
  Bottom 0.406: Q14.3 30,22.25 V2.9
N$38
  Bottom 0.406: Q15.3 30,32.25 V2.8
N$39
  Bottom 0.406: Q16.3 33.5,34 V2.7
N$40
  Bottom 0.406: Q17.3 37,35.5 V2.6
N$41
  Bottom 0.406: Q18.3 40.5,35 V2.5
N$42
  Bottom 0.406: V2.4 44.25,36.65 Q19.3
N$43
  Bottom 0.406: V2.3 44.25,24.75 40,20.5 40,15 40.5,14.5 Q20.3
N$44
  Bottom 0.406: R14.2 38.05,8.4 38.05,10.8 Q12.1
N$45
  Bottom 0.406: R15.2 34.55,8.4 34.55,10.8 Q13.1
N$46
  Bottom 0.406: R16.2 31.05,8.4 31.05,10.8 Q14.1
N$47
  Bottom 0.406: R17.2 28.95,41.1 28.95,39.1 Q15.1
N$48
  Bottom 0.406: R18.2 32.45,41.1 32.45,39.1 Q16.1
N$49
  Bottom 0.406: R19.2 35.95,41.1 35.95,39.1 Q17.1
N$50
  Bottom 0.406: R20.2 39.45,41.1 39.45,39.1 Q18.1
N$51
  Bottom 0.406: R21.2 42.95,41.1 42.95,39.1 Q19.1
N$52
  Bottom 0.406: R22.2 41.55,8.4 41.55,10.8 Q20.1
N$53
  Bottom 0.406: R13.2 45.05,8.4 45.05,10.8 Q11.1
N$54
  Bottom 0.406: SV1.7 28.27,3.77 29.5,5 30.5,5 31,5.5 R16.1
N$55
  Bottom 0.406: SV1.8 30.81,3.81 33.5,6.5 34.35,6.5 R15.1
N$56
  Bottom 0.406: SV1.9 33.35,3.85 34.5,5 35.5,5 37,6.5 37.85,6.5 R14.1
N$57
  Bottom 0.406: SV1.10 35.89,3.89 37.5,5.5 39,5.5 40,6.5 41.35,6.5 R22.1
N$58
  Bottom 0.406: SV1.11 38.43,3.93 39,4.5 39.5,4.5 40,5 44.5,5 45,5.5 R13.1
N$59  (via drill 0.6)
  Top 0.406: v27,6.5 39.5,6.5 41,5 41,2.53 SV1.12
  Bottom 0.406: SV1.12 45,2.5 49.25,6.75 R12.1 R67.2 | R1.1 25.25,7.5 26.25,6.5 v27,6.5
N$60
  Bottom 0.406: SV2.7 28.27,45.23 29,44.5 R17.1
N$61
  Bottom 0.406: 32.35,43 R18.1 32.5,44 30.81,45.69 SV2.8
N$62
  Bottom 0.406: SV2.9 33.35,45.65 34.5,44.5 35.5,44.5 36,44 R19.1
N$63
  Bottom 0.406: SV2.10 35.89,46.11 37,45 38.5,45 39.5,44 R20.1
N$64
  Bottom 0.406: SV2.11 38.43,47.07 40.5,45 42.5,45 43,44.5 R21.1
N$65
  Bottom 0.406: V3.1 76.5,17 78.5,15 R23.2
N$66
  Bottom 0.406: V3.2 73,20.5 71,18.5 71,15.5 71.5,15 73.5,15 74,14.5 Q21.3
N$67
  Bottom 0.406: Q22.3 67,16 66,17 V3.11
N$68
  Bottom 0.406: Q23.3 63.5,14.5 62.75,15.25 V3.10
N$69
  Bottom 0.406: Q24.3 60,22.25 V3.9
N$70
  Bottom 0.406: V3.8 62.75,29.75 60,32.5 Q25.3
N$71
  Bottom 0.406: V3.7 63.5,34 Q26.3
N$72
  Bottom 0.406: V3.6 67,35.5 Q27.3
N$73
  Bottom 0.406: V3.5 70.5,35 Q28.3
N$74
  Bottom 0.406: V3.4 74.25,36.65 Q29.3
N$75
  Bottom 0.406: V3.3 74,25 70,21 70,15 70.5,14.5 Q30.3
N$76
  Bottom 0.406: R25.2 68.05,8.4 68.05,10.8 Q22.1
N$77
  Bottom 0.406: R26.2 64.55,8.4 64.55,10.8 Q23.1
N$78
  Bottom 0.406: R27.2 61.05,8.4 61.05,10.8 Q24.1
N$79
  Bottom 0.406: R28.2 58.95,41.1 58.95,39.1 Q25.1
N$80
  Bottom 0.406: R29.2 62.45,41.1 62.45,39.1 Q26.1
N$81
  Bottom 0.406: R30.2 65.95,41.1 65.95,39.1 Q27.1
N$82
  Bottom 0.406: R31.2 69.45,41.1 69.45,39.1 Q28.1
N$83
  Bottom 0.406: R32.2 72.95,41.1 72.95,39.1 Q29.1
N$84
  Bottom 0.406: R33.2 71.55,8.4 71.55,10.8 Q30.1
N$85
  Bottom 0.406: R24.2 75.05,8.4 75.05,10.8 Q21.1
N$86
  Bottom 0.406: SV3.1 64,2.5 61,5.5 R27.1
N$87
  Bottom 0.406: SV3.2 68.57,3.93 67.5,5 65,5 64.5,5.5 R26.1
N$88
  Bottom 0.406: SV3.3 71.11,3.89 69.5,5.5 68.5,5.5 68,6 R25.1
N$89
  Bottom 0.406: SV3.4 73.65,3.35 71.5,5.5 R33.1
N$90
  Bottom 0.406: SV3.5 76.19,3.81 75,5 R24.1
N$91  (via drill 0.6)
  Top 0.305: IC2.9 32.05,79.31 v32,79.25 | v14.75,79.25 14.75,71.25 15.6,70.41 IC3.14
  Bottom 0.305: v32,79.25 v14.75,79.25
N$92
  Bottom 0.406: SV4.1 61.5,47.5 59,45 R28.1
N$93
  Bottom 0.406: SV4.2 68.57,46.57 67,45 63,45 62.5,44.5 R29.1
N$94
  Bottom 0.406: SV4.3 71.11,46.61 68.5,44 66.5,44 66,43.5 R30.1
N$95
  Bottom 0.406: SV4.4 73.65,46.65 71,44 71,43.5 70.5,43 69.65,43 R31.1
N$96
  Bottom 0.406: SV4.5 76.19,47.19 73,44 R32.1
N$97
  Bottom 0.406: V4.1 99.5,17 101.5,15 R34.2
N$98
  Bottom 0.406: V4.2 96,20.5 94,18.5 94,15.5 94.5,15 96.5,15 97,14.5 Q31.3
N$99
  Bottom 0.406: V4.11 89,17 90,16 Q32.3
N$100
  Bottom 0.406: V4.10 85.75,15.25 86.5,14.5 Q33.3
N$101
  Bottom 0.406: Q34.3 83,22.25 V4.9
N$102
  Bottom 0.406: Q35.3 83,32.25 V4.8
N$103
  Bottom 0.406: Q36.3 86.5,34 V4.7
N$104
  Bottom 0.406: Q37.3 90,35.5 V4.6
N$105
  Bottom 0.406: Q38.3 93.5,35 V4.5
N$106
  Bottom 0.406: V4.4 97.25,36.65 Q39.3
N$107
  Bottom 0.406: V4.3 97.25,24.75 93,20.5 93,15 93.5,14.5 Q40.3
N$108
  Bottom 0.406: R36.2 91.05,8.4 91.05,10.8 Q32.1
N$109
  Bottom 0.406: R37.2 87.55,8.4 87.55,10.8 Q33.1
N$110
  Bottom 0.406: R38.2 84.05,8.4 84.05,10.8 Q34.1
N$111
  Bottom 0.406: R39.2 81.95,41.1 81.95,39.1 Q35.1
N$112
  Bottom 0.406: R40.2 85.45,41.1 85.45,39.1 Q36.1
N$113
  Bottom 0.406: R41.2 88.95,41.1 88.95,39.1 Q37.1
N$114
  Bottom 0.406: R42.2 92.45,41.1 92.45,39.1 Q38.1
N$115
  Bottom 0.406: R43.2 95.95,41.1 95.95,39.1 Q39.1
N$116
  Bottom 0.406: R44.2 94.55,8.4 94.55,10.8 Q40.1
N$117
  Bottom 0.406: R35.2 98.05,8.4 98.05,10.8 Q31.1
N$118
  Bottom 0.406: SV3.7 81.27,3.77 82.5,5 83.5,5 84,5.5 R38.1
N$119
  Bottom 0.406: SV3.8 83.81,3.81 86.5,6.5 87.35,6.5 R37.1
N$120
  Bottom 0.406: SV3.9 86.35,3.85 87.5,5 88.5,5 90,6.5 90.85,6.5 R36.1
N$121
  Bottom 0.406: SV3.10 88.89,3.89 90.5,5.5 92,5.5 93,6.5 94.35,6.5 R44.1
N$122
  Bottom 0.406: SV3.11 91.43,3.93 92,4.5 92.5,4.5 93,5 97.5,5 98,5.5 R35.1
N$123  (via drill 0.6)
  Top 0.305: IC10.20 59.65,72.6 v60,72.25 | v60,74.5 60.75,75.25 60.75,76 61.25,76.5 61.9,76.5 C17.1
  Bottom 0.305: v60,72.25 v60,74.5
N$124
  Bottom 0.406: SV4.7 81.27,45.23 82,44.5 R39.1
N$125
  Bottom 0.406: 85.35,43 R40.1 85.5,44 83.81,45.69 SV4.8
N$126
  Bottom 0.406: SV4.9 86.35,45.65 87.5,44.5 88.5,44.5 89,44 R41.1
N$127
  Bottom 0.406: SV4.10 88.89,46.11 90,45 91.5,45 92.5,44 R42.1
N$128
  Bottom 0.406: SV4.11 91.43,47.07 93.5,45 95.5,45 96,44.5 R43.1
N$129
  Bottom 0.406: V5.1 129.5,17 131.5,15 R45.2
N$130
  Bottom 0.406: V5.2 126,20.5 124,18.5 124,15.5 124.5,15 126.5,15 127,14.5 Q41.3
N$131
  Bottom 0.406: Q42.3 120,16 119,17 V5.11
N$132
  Bottom 0.406: Q43.3 116.5,14.5 115.75,15.25 V5.10
N$133
  Bottom 0.406: Q44.3 113,22.25 V5.9
N$134
  Bottom 0.406: V5.8 115.75,29.75 113,32.5 Q45.3
N$135
  Bottom 0.406: V5.7 116.5,34 Q46.3
N$136
  Bottom 0.406: V5.6 120,35.5 Q47.3
N$137
  Bottom 0.406: V5.5 123.5,35 Q48.3
N$138
  Bottom 0.406: V5.4 127.25,36.65 Q49.3
N$139
  Bottom 0.406: V5.3 127,25 123,21 123,15 123.5,14.5 Q50.3
N$140
  Bottom 0.406: R47.2 121.05,8.4 121.05,10.8 Q42.1
N$141
  Bottom 0.406: R48.2 117.55,8.4 117.55,10.8 Q43.1
N$142
  Bottom 0.406: R49.2 114.05,8.4 114.05,10.8 Q44.1
N$143
  Bottom 0.406: R50.2 111.95,41.1 111.95,39.1 Q45.1
N$144
  Bottom 0.406: R51.2 115.45,41.1 115.45,39.1 Q46.1
N$145
  Bottom 0.406: R52.2 118.95,41.1 118.95,39.1 Q47.1
N$146
  Bottom 0.406: R53.2 122.45,41.1 122.45,39.1 Q48.1
N$147
  Bottom 0.406: R54.2 125.95,41.1 125.95,39.1 Q49.1
N$148
  Bottom 0.406: R55.2 124.55,8.4 124.55,10.8 Q50.1
N$149
  Bottom 0.406: R46.2 128.05,8.4 128.05,10.8 Q41.1
N$150
  Bottom 0.406: SV5.1 117,2.5 114,5.5 R49.1
N$151
  Bottom 0.406: SV5.2 121.57,3.93 120.5,5 118,5 117.5,5.5 R48.1
N$152
  Bottom 0.406: SV5.3 124.11,3.89 122.5,5.5 121.5,5.5 121,6 R47.1
N$153
  Bottom 0.406: SV5.4 126.65,3.35 124.5,5.5 R55.1
N$154
  Bottom 0.406: SV5.5 129.19,3.81 128,5 R46.1
N$155
  Top 0.305: IC10.29 53.35,84.9 51.71,86.54 | SV14.5 51.71,90.25 | 51.71,90.25 51.71,86.54 | 51.71,86.5 51.71,86.54 | C9.1 R71.1 51.48,90.35 arc-45 51.7,90.26 51.71,90.25
N$156
  Bottom 0.406: SV6.1 114.5,47.5 112,45 R50.1
N$157
  Bottom 0.406: SV6.2 121.57,46.57 120,45 116,45 115.5,44.5 R51.1
N$158
  Bottom 0.406: SV6.3 124.11,46.61 121.5,44 119.5,44 119,43.5 R52.1
N$159
  Bottom 0.406: SV6.4 126.65,46.65 124,44 124,43.5 123.5,43 122.65,43 R53.1
N$160
  Bottom 0.406: SV6.5 129.19,47.19 126,44 R54.1
N$161
  Bottom 0.406: V6.1 152.75,17 154.75,15 R56.2
N$162
  Bottom 0.406: V6.2 149,20.5 147,18.5 147,15.5 147.5,15 149.5,15 150,14.5 Q51.3
N$163
  Bottom 0.406: V6.11 142,17 143,16 Q52.3
N$164
  Bottom 0.406: V6.10 138.75,15.25 139.5,14.5 Q53.3
N$165
  Bottom 0.406: Q54.3 136,22.25 V6.9
N$166
  Bottom 0.406: Q55.3 136,32.25 V6.8
N$167
  Bottom 0.406: Q56.3 139.5,34 V6.7
N$168
  Bottom 0.406: Q57.3 143,35.5 V6.6
N$169
  Bottom 0.406: Q58.3 146.5,35 V6.5
N$170
  Bottom 0.406: V6.4 150.25,36.65 Q59.3
N$171
  Bottom 0.406: V6.3 150.25,24.75 146,20.5 146,15 146.5,14.5 Q60.3
N$172
  Bottom 0.406: R58.2 144.05,8.4 144.05,10.8 Q52.1
N$173
  Bottom 0.406: R59.2 140.55,8.4 140.55,10.8 Q53.1
N$174
  Bottom 0.406: R60.2 137.05,8.4 137.05,10.8 Q54.1
N$175
  Bottom 0.406: R61.2 134.95,41.1 134.95,39.1 Q55.1
N$176
  Bottom 0.406: R62.2 138.45,41.1 138.45,39.1 Q56.1
N$177
  Bottom 0.406: R63.2 141.95,41.1 141.95,39.1 Q57.1
N$178
  Bottom 0.406: R64.2 145.45,41.1 145.45,39.1 Q58.1
N$179
  Bottom 0.406: R65.2 148.95,41.1 148.95,39.1 Q59.1
N$180
  Bottom 0.406: R66.2 147.55,8.4 147.55,10.8 Q60.1
N$181
  Bottom 0.406: R57.2 151.05,8.4 151.05,10.8 Q51.1
N$182
  Bottom 0.406: SV5.7 134.27,3.77 135.5,5 136.5,5 137,5.5 R60.1
N$183
  Bottom 0.406: SV5.8 136.81,3.81 139.5,6.5 140.35,6.5 R59.1
N$184
  Bottom 0.406: SV5.9 139.35,3.85 140.5,5 141.5,5 143,6.5 143.85,6.5 R58.1
N$185
  Bottom 0.406: SV5.10 141.89,3.89 143.5,5.5 145,5.5 146,6.5 147.35,6.5 R66.1
N$186
  Bottom 0.406: SV5.11 144.43,3.93 145,4.5 145.5,4.5 146,5 150.5,5 151,5.5 R57.1
N$187  (via drill 0.6)
  Top 0.406: v133,6.5 145.5,6.5 147,5 147,2.53 SV5.12
  Bottom 0.406: SV5.12 152.75,2.5 154.75,4.5 R56.1 | R45.1 131.5,7.5 132.5,6.5 v133,6.5
N$188
  Bottom 0.406: SV6.7 134.27,45.23 135,44.5 R61.1
N$189
  Bottom 0.406: 138.35,43 R62.1 138.5,44 136.81,45.69 SV6.8
N$190
  Bottom 0.406: SV6.9 139.35,45.65 140.5,44.5 141.5,44.5 142,44 R63.1
N$191
  Bottom 0.406: SV6.10 141.89,46.11 143,45 144.5,45 145.5,44 R64.1
N$192
  Bottom 0.406: SV6.11 144.43,47.07 146.5,45 148.5,45 149,44.5 R65.1
N$193  (via drill 0.6)
  Top 0.406: v80,6.5 92,6.5 94,4.5 94,2.53 SV3.12
  Bottom 0.406: SV3.12 99.5,2.5 101.5,4.5 R34.1 R68.2 | R23.1 78.5,7.5 79.5,6.5 v80,6.5
N$194
  Bottom 0.406: LMP1.C 54.77,27.23 47.5,34.5 Q61.3
N$195
  Bottom 0.305: R67.1 53.5,20.75 52.25,22 52.25,24.98 LMP1.A
N$196
  Bottom 0.406: Q61.1 46.55,41.1 R69.1
N$197
  Bottom 0.406: SV2.12 43.5,47.5 46.5,44.5 R69.2
N$198
  Bottom 0.305: R68.1 105.75,22.25 105.25,22.75 105.25,24.98 LMP2.A
N$199
  Bottom 0.406: LMP2.C 107.77,25.98 106.5,27.25 100.75,27.25 99.75,28.25 99.75,35 100.5,35.75 Q62.3
N$200
  Bottom 0.406: R70.1 99.5,39.15 Q62.1
N$201
  Bottom 0.406: SV4.12 97,47.5 99.5,45 R70.2
N$202
  Bottom 0.406: IC11.1 102.75,35.75 103.4,36.4 C11.2 103.4,47.44 SV13.1
N$203
  Top 0.305: IC1.7 13.32,94.42 13,94.75 13,98.47 SV8.1
N$204
  Top 0.305: IC1.6 14.6,96.59 15.5,97.5 15.5,98.43 SV8.2
N$205
  Top 0.305: IC1.5 15.87,95.86 18,98 18,98.39 SV8.3
N$206
  Top 0.305: IC1.4 17.14,95.39 18,96.25 19.25,96.25 20.75,97.75 20.75,98.4 SV8.4
N$207
  Top 0.305: IC1.3 18.41,95.16 18.75,95.5 21,95.5 23.25,97.75 23.25,98.44 SV8.5
N$208
  Top 0.305: IC1.2 19.68,94.17 20.25,94.75 22.25,94.75 23.75,96.25 27,96.25 28.25,97.5 28.25,98.48 SV8.7
N$209
  Top 0.305: IC1.1 20.95,93.69 21.25,94 22.75,94 24.25,95.5 28.75,95.5 30.75,97.5 30.75,98.44 SV8.8
N$210
  Top 0.305: IC2.7 33.33,98.47 SV8.9
N$211
  Top 0.305: IC2.6 34.59,96.09 36,97.5 36,98.39 SV8.10
N$212
  Top 0.305: IC2.5 35.87,95.11 38.5,97.75 38.5,98.43 SV8.11
N$213
  Top 0.305: IC2.4 37.13,94.89 38.75,96.5 39.75,96.5 41,97.75 41,98.47 SV8.12
N$214
  Top 0.305: IC3.1 13.05,53.52 SV7.1
N$215
  Top 0.305: IC3.2 14.32,57.17 15.5,56 15.5,53.57 SV7.2
N$216
  Top 0.305: IC3.3 15.6,57.16 17,55.75 17.5,55.75 18,55.25 18,53.61 SV7.3
N$217
  Top 0.305: IC3.4 16.86,57.38 18,56.25 18.5,56.25 20.5,54.25 20.5,53.65 SV7.4
N$218
  Top 0.305: IC3.5 18.14,57.87 20.25,55.75 21.5,55.75 23.19,54.06 SV7.5
N$219
  Top 0.305: IC3.6 19.41,57.84 20.5,56.75 22,56.75 23,55.75 27.75,55.75 28.25,55.25 28.25,53.52 SV7.7
N$220
  Top 0.305: IC3.7 20.68,58.08 21,57.75 22.75,57.75 24,56.5 30,56.5 30.75,55.75 30.75,53.56 SV7.8
N$221
  Top 0.305: IC2.1 41.93,92.57 42.5,92 42.5,84 36.5,78 20.75,78 19.75,77 19.75,72.75 26.25,66.25 26.25,60 28.25,58 31,58 33.25,55.75 33.25,53.6 SV7.9
N$222
  Top 0.305: IC2.2 39.67,94.42 40,94.75 42.25,94.75 43.25,93.75 43.25,83.75 36.75,77.25 21.25,77.25 20.5,76.5 20.5,73.25 27,66.75 27,60.5 28.75,58.75 31.75,58.75 36,54.5 36,53.61 SV7.10
N$223
  Top 0.305: IC2.3 38.41,94.91 39,95.5 42.75,95.5 44,94.25 44,83.25 37.25,76.5 21.75,76.5 21.25,76 21.25,73.75 27.75,67.25 27.75,60.75 29,59.5 34,59.5 38.5,55 38.5,53.57 SV7.11
N$224  (via drill 0.6)
  Top 0.305: IC5.14 91.41,83.66 v89.75,82 | IC4.9 65.06,82.19 v65.25,82
  Bottom 0.305: v89.75,82 v65.25,82
N$225  (via drill 0.6)
  Top 0.305: IC6.14 68.59,79.09 v68.75,79.25 | IC5.9 85.06,80.81 v85,80.75
  Bottom 0.305: v68.75,79.25 71.75,79.25 73.25,80.75 v85,80.75
N$226
  Bottom 0.406: IC11.2 105.25,34.55 105.25,35.75 105.1,35.9 C11.1 105.1,39.75 R75.2
N$227
  Bottom 0.406: IC11.3 110.25,34.5 108.5,36.25 108.5,47.46 SV13.3
N$228  (via drill 0.6)
  Top 0.305: IC4.14 71.41,80.66 v71.25,80.5 | v18.25,80.5 18.25,72.75 22,69 22,66.25 21.95,66.19 IC3.9
  Bottom 0.305: v71.25,80.5 54.25,80.5 52.5,78.75 44.75,78.75 43,80.5 v18.25,80.5
N$229
  Top 0.305: IC4.7 66.33,94.92 66,95.25 66,98.47 SV10.1
N$230
  Top 0.305: IC4.6 67.59,94.34 68.5,95.25 68.5,98.43 SV10.2
N$231
  Top 0.305: IC4.5 68.86,94.36 71,96.5 71,98.39 SV10.3
N$232
  Top 0.305: IC4.4 70.14,94.39 73.5,97.75 73.5,98.35 SV10.4
N$233
  Top 0.305: IC4.3 71.41,94.16 73.5,96.25 75.75,96.25 76.25,96.75 76.25,98.44 SV10.5
N$234
  Top 0.305: IC4.2 72.67,94.17 73.75,95.25 79.75,95.25 81.25,96.75 81.25,98.48 SV10.7
N$235
  Top 0.305: IC4.1 73.94,93.69 74.5,94.25 82,94.25 83.75,96 83.75,98.44 SV10.8
N$236
  Top 0.305: IC5.7 86.33,98.47 SV10.9
N$237
  Top 0.305: IC5.6 87.59,93.84 89,95.25 89,98.39 SV10.10
N$238
  Top 0.305: IC5.5 88.86,94.11 91.5,96.75 91.5,98.43 SV10.11
N$239
  Top 0.305: IC5.4 90.14,94.39 93.75,98 93.75,98.28 SV10.12
N$240
  Top 0.305: IC6.1 66.06,53.52 SV9.1
N$241
  Top 0.305: IC6.2 67.33,55.42 68.5,54.25 68.5,53.57 SV9.2
N$242
  Top 0.305: IC6.3 68.59,56.16 69,55.75 69.75,55.75 71,54.5 71,53.61 SV9.3
N$243
  Top 0.305: IC6.4 69.86,56.88 71,55.75 72,55.75 73.5,54.25 73.5,53.65 SV9.4
N$244
  Top 0.305: IC6.5 71.14,57.12 71.5,56.75 72.25,56.75 73.25,55.75 74.5,55.75 76,54.25 76,53.69 SV9.5
N$245
  Top 0.305: IC6.6 72.41,57.84 73.25,57 74.75,57 76,55.75 79.75,55.75 81.25,54.25 81.25,53.52 SV9.7
N$246
  Top 0.305: IC6.7 73.67,58.08 74,57.75 75.25,57.75 76.25,56.75 81.25,56.75 83.75,54.25 83.75,53.56 SV9.8
N$247
  Top 0.305: IC5.1 94.93,92.57 95.5,92 95.5,85.75 88,78.25 74.5,78.25 73,76.75 73,70.75 78.75,65 78.75,60.5 81,58.25 83.5,58.25 86.25,55.5 86.25,53.6 SV9.9
N$248
  Top 0.305: IC5.2 92.67,93.92 93,94.25 95,94.25 96.25,93 96.25,85.5 88,77.25 75,77.25 74,76.25 74,71 79.5,65.5 79.5,61 81.5,59 84.5,59 89,54.5 89,53.61 SV9.10
N$249
  Top 0.305: IC5.3 91.41,94.41 92,95 95.25,95 97,93.25 97,85.25 88.25,76.5 75.75,76.5 75,75.75 75,71.25 80.25,66 80.25,61.5 82,59.75 87.25,59.75 91.5,55.5 91.5,53.57 SV9.11
N$250  (via drill 0.6)
  Top 0.305: IC8.14 118.41,74.66 v117.75,74 | IC7.9 99.06,74.19 v99.25,74
  Bottom 0.305: v117.75,74 v99.25,74
N$251  (via drill 0.6)
  Top 0.305: IC9.14 103.09,72.09 v103.75,72.75 | IC8.9 112.06,73.31 v111.5,72.75
  Bottom 0.305: v111.5,72.75 v103.75,72.75
N$252
  Bottom 0.406: R75.1 105.25,43.75 106,44.5 SV13.2
N$253
  Top 0.305: IC12.1 IC12.8 IC12.7 126.36,67.61 127,68.25 127,73 127.5,73.5 R76.1
  Top 0.61: R76.1 128.83,76.83 130.5,78.5 136.25,78.5 138,76.75 L1.1
N$254  (via drill 0.6)
  Top 0.305: IC6.9 74.94,67.56 72.25,70.25 72.25,78.25 73.5,79.5 v74.75,79.5 | IC7.14 105.41,76.66 v101.5,72.75
  Bottom 0.305: v74.75,79.5 85.5,79.5 86.5,80.5 91,80.5 98.75,72.75 v101.5,72.75
N$255
  Top 0.305: IC7.7 100.33,86.33 109.5,95.5 118,95.5 119,96.5 119,98.47 SV12.1
N$256
  Top 0.305: SV12.2 121.5,98.43 121.5,96 120.25,94.75 109.75,94.75 101.59,86.59 IC7.6
N$257
  Top 0.305: SV12.3 124.25,98.36 124.25,96 122.25,94 110,94 102.86,86.86 IC7.5
N$258
  Top 0.305: SV12.4 126.75,98.4 126.75,96 124,93.25 110.25,93.25 104.14,87.14 IC7.4
N$259
  Top 0.305: SV12.5 129.25,98.44 129.25,95.75 126,92.5 110.5,92.5 105.41,87.41 IC7.3
N$260
  Top 0.305: SV12.7 134.25,98.48 134.25,96.75 129.25,91.75 110.75,91.75 106.67,87.67 IC7.2
N$261
  Top 0.305: IC7.1 107.94,87.69 111.25,91 129.5,91 136.81,98.31 SV12.8
N$262
  Top 0.305: IC8.7 113.33,89.08 114.5,90.25 129.75,90.25 135.75,96.25 138,96.25 139.35,97.6 SV12.9
N$263
  Top 0.305: IC8.6 114.59,88.84 115.25,89.5 130,89.5 136,95.5 140.5,95.5 141.89,96.89 SV12.10
N$264
  Top 0.305: IC8.5 115.86,88.11 116.5,88.75 130.25,88.75 136.25,94.75 142.25,94.75 144.43,96.93 SV12.11
N$265
  Top 0.305: IC8.4 117.14,87.64 117.5,88 130.5,88 136.5,94 143.75,94 146.97,97.22 SV12.12
N$266
  Top 0.305: 119.06,53.52 SV11.1 119,53.53 119,55.25 118.25,56 103.5,56 100.56,58.95 IC9.1
N$267
  Top 0.305: SV11.2 121.5,53.57 121.5,54 121.5,54.25 121.5,55.5 120.25,56.75 103.75,56.75 101.83,58.67 IC9.2
N$268
  Top 0.305: IC9.3 103.09,58.66 104.25,57.5 122.25,57.5 124,55.75 124,53.61 SV11.3
N$269
  Top 0.305: IC9.4 104.36,58.88 105,58.25 124.5,58.25 126.75,56 126.75,53.6 SV11.4
N$270
  Top 0.305: IC9.5 105.64,59.87 106.5,59 126,59 129.25,55.75 129.25,53.56 SV11.5
N$271
  Top 0.305: IC9.6 106.91,60.34 107.5,59.75 127.5,59.75 131.5,55.75 133.75,55.75 134.25,55.25 134.25,53.52 SV11.7
N$272
  Top 0.305: IC9.7 108.17,61.08 108.75,60.5 127.75,60.5 131.75,56.5 134,56.5 134.75,55.75 136.5,55.75 136.75,55.5 136.75,53.56 SV11.8
N$273
  Top 0.305: IC8.1 121.93,84.57 122.25,84.25 122.25,76.5 118.5,72.75 114.25,72.75 113,71.5 113,62 113.75,61.25 128,61.25 132,57.25 134.25,57.25 135,56.5 136.75,56.5 137.5,55.75 139.25,55.75 139.5,55.5 139.5,53.65 SV11.9
N$274
  Top 0.305: IC8.2 119.67,86.17 120,86.5 122,86.5 123,85.5 123,76.25 118.75,72 114.75,72 113.75,71 113.75,62.5 114.25,62 128.25,62 132.25,58 134.5,58 135.25,57.25 137,57.25 137.75,56.5 139.5,56.5 140.25,55.75 141.75,55.75 142,55.5 142,53.61 SV11.10
N$275
  Top 0.305: IC8.3 118.41,86.41 119.25,87.25 122.75,87.25 123.75,86.25 123.75,75.75 119.25,71.25 115.25,71.25 114.5,70.5 114.5,63.25 115,62.75 128.5,62.75 132.5,58.75 134.75,58.75 135.5,58 137.25,58 138,57.25 139.75,57.25 140.5,56.5 142,56.5 142.75,55.75 144.25,55.75 144.5,55.5 144.5,53.57 SV11.11
N$276
  Top 0.305: Q63.B D2.A 134.75,66.5 133.63,67.61 133.5,67.61 | IC12.2 133.5,67.61 | R80.1 133.5,67.61
N$277
  Top 0.305: IC12.3 131.99,68.89 C12.1
N$278
  Top 1.27: L1.2 149.5,76.75 149.5,66.25 | 149.5,66.25 149,66.25 T1.3 | 149.5,64.28 149.5,64.5 | 149.5,64.5 149.5,66.25 | D1.A 151,60.75 151,64.5 149.5,64.5
N$279  (via drill 0.6)
  Top 0.305: R77.1 134.5,60.75 130.5,64.75 122.75,64.75 122,65.5 122,70.16 | IC12.5 123,70.16 | 123,70.16 122,70.16 | 122,70.16 121.59,70.16 v121.25,70.5 | v59.75,78 59.75,75.75 59,75 IC10.23 | 123,70.16 123,71.9 R78.2
  Bottom 0.305: v121.25,70.5 111.75,70.5 111,71.25 98.75,71.25 92,78 v59.75,78
N$280
  Top 0.305: Q63.E D2.C 139.65,66.5 R79.2
N$281
  Top 0.305: R79.1 141.52,68.1 T1.1
N$282  (via drill 0.6)
  Top 0.305: v83.5,92.5 v83.5,86 | v46,85.5 46,83.25 41.25,78.5 v41.25,77.75 | IC10.11 52.55,70.2 v52.25,70.5
  Bottom 0.305: SV15.3 108.54,97.29 103.75,92.5 v83.5,92.5 | v83.5,86 59,86 58.25,85.25 46.25,85.25 v46,85.5 | v52.25,70.5 52.25,71.5 46,77.75 v41.25,77.75
N$283
  Top 0.305: IC10.30 52.55,79.7 TP1.TP
N$284
  Top 0.305: IC10.31 51.75,78.5 51.5,78.75 50.5,78.75 TP2.TP
N$285
  Top 0.305: IC14.9 IC14.10 IC14.5
N$287
  Top 0.305: IC10.10 51.75,66.75 48.5,63.5 48.5,59 48.9,58.6 IC13.4 52.4,58.6 52.75,58.25 52.75,57.15 R73.1
N$288
  Top 0.305: IC14.4 86.25,63.75 86,63.5 83.71,63.5 | IC14.2 83.71,63.5 | 83.71,63.5 83.71,61.54 TP4.TP
N$289
  Top 0.305: IC10.7 46.27,71 Q64.2 44.98,71.27 44.5,71.75 44.5,72.6 C15.1
N$290
  Top 0.305: IC10.8 47.47,70.2 Q64.1 46,67.75 45.5,67.25 C16.1
N$291
  Top 0.305: TP5.TP 88.79,61.71 IC14.6 88.79,68.54 90.06,69.81 IC14.8
N$292  (via drill 0.6)
  Top 0.305: IC14.1 82.44,66.69 | 82.44,66.69 82.75,67 84.75,67 | IC14.3 84.98,66.77 84.75,67 | 84.75,67 86.25,68.5 IC14.11 | IC10.13 54.15,67.65 53.5,67 v53.25,67 | v80.5,67.5 81.25,66.75 82.38,66.75 82.44,66.69
  Bottom 0.305: v53.25,67 54.75,68.5 67.5,68.5 68,69 70.5,69 71,68.5 79.5,68.5 v80.5,67.5
SCK  (via drill 0.6)
  Top 0.305: IC1.11 14.6,83.41 v14.75,83.25 | IC5.11 87.59,84.09 v86.75,83.25 | IC4.11 67.59,83.34 v67.5,83.25 | IC2.11 34.59,83.34 v34.5,83.25 | IC8.11 114.59,75.41 v114.75,75.25 | IC7.11 101.59,75.34 v101.5,75.25 | IC3.11 19.41,70.09 17,72.5 17,83 v17.25,83.25 | 72.41,83.16 v72.5,83.25 72.5,80 71.25,78.75 v71.25,70 72.41,68.84 IC6.11 | SV14.3 54.27,94.98 55.75,93.5 v55.75,83.25 | IC13.2 53.4,61.15 58.25,66 58.25,69.86 arc45 58.16,70.09 IC10.17 60.05,70.2 v60.5,69.75 | IC9.11 106.91,73.41 v108.75,75.25
  Bottom 0.305: v14.75,83.25 v17.25,83.25 v34.5,83.25 v55.75,83.25 v67.5,83.25 v72.5,83.25 v86.75,83.25 91.75,83.25 92,83 92,81 97.75,75.25 v101.5,75.25 v108.75,75.25 v114.75,75.25 | v71.25,70 67.75,70 67.5,69.75 v60.5,69.75
V+
  Top 0.305: SV11.12 150.25,53.5 154,57.25 | D1.C 155.28,58.52 154,57.25 | R77.2 147.92,58.33 148.5,57.75 153.5,57.75 154,57.25
  Top 1.27: C13.1 156.01,66.76 155.25,66 155.25,60.77 D1.C
  Bottom 0.305: SV7.12 40.97,54.47 42.75,56.25 92.25,56.25 94,54.5 94,53.53 SV9.12 93.97,54.72 95.5,56.25 145.5,56.25 147,54.75 147,53.53 SV11.12
(copper drawn outside any net)
  shapes: Top circle x1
